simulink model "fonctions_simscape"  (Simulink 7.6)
settings: Solver=ode15s  StartTime=0.0  StopTime=1  RelTol=1e-3
InitFcn:
  | R1=10e3;
  | R2=20e3;
libraries: fl_lib x12, nesl_utility x4, elec_lib x1

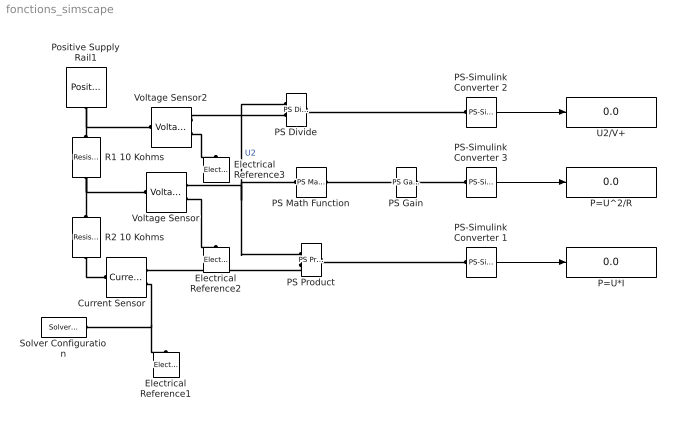
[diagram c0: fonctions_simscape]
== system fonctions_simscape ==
  Current Sensor : fl_lib/Electrical/Electrical Sensors/Current Sensor  DialogController=NetworkEngine.DynNeDlgSource  SystemSampleTime=-1  i1_Log=off  v1_Log=off  LocalVarNames=|i1|v1  LocalVarDescs=|i1|v1  LocalVarLogging=[0 0]
  Electrical Reference1 : fl_lib/Electrical/Electrical Elements/Electrical Reference  DialogController=NetworkEngine.DynNeDlgSource  SystemSampleTime=-1  i_Log=off  LocalVarNames=|i  LocalVarDescs=|i  LocalVarLogging=[]
  Electrical Reference2 : fl_lib/Electrical/Electrical Elements/Electrical Reference  DialogController=NetworkEngine.DynNeDlgSource  SystemSampleTime=-1  i_Log=off  LocalVarNames=|i  LocalVarDescs=|i  LocalVarLogging=[]
  Electrical Reference3 : fl_lib/Electrical/Electrical Elements/Electrical Reference  DialogController=NetworkEngine.DynNeDlgSource  SystemSampleTime=-1  i_Log=off  LocalVarNames=|i  LocalVarDescs=|i  LocalVarLogging=[]
  P=U*I : Display
  P=U^2/R : Display
  PS Divide : fl_lib/Physical Signals/Functions/PS Divide  DialogController=NetworkEngine.DynNeDlgSource  SystemSampleTime=-1  LocalVarLogging=[]
  PS Gain : fl_lib/Physical Signals/Functions/PS Gain  DialogController=NetworkEngine.DynNeDlgSource  SystemSampleTime=-1  gain=1/R2  LocalVarLogging=[]
  PS Math Function : fl_lib/Physical Signals/Functions/PS Math Function  DialogController=NetworkEngine.DynNeDlgSource  SystemSampleTime=-1  fcn_choice=7  LocalVarLogging=[]
  PS Product : fl_lib/Physical Signals/Functions/PS Product  DialogController=NetworkEngine.DynNeDlgSource  SystemSampleTime=-1  LocalVarLogging=[]
  PS-Simulink Converter 1 : nesl_utility/PS-Simulink Converter  DialogController=NetworkEngine.DynNeUtilDlgSource  SystemSampleTime=-1  PhysicalDomain=network_engine_domain  LeftPortType=input  RightPortType=output  SubClassName=ps_output  Unit=W  AffineConversion=off
  PS-Simulink Converter 2 : nesl_utility/PS-Simulink Converter  DialogController=NetworkEngine.DynNeUtilDlgSource  SystemSampleTime=-1  PhysicalDomain=network_engine_domain  LeftPortType=input  RightPortType=output  SubClassName=ps_output  Unit=V  AffineConversion=off
  PS-Simulink Converter 3 : nesl_utility/PS-Simulink Converter  DialogController=NetworkEngine.DynNeUtilDlgSource  SystemSampleTime=-1  PhysicalDomain=network_engine_domain  LeftPortType=input  RightPortType=output  SubClassName=ps_output  Unit=W  AffineConversion=off
  Positive Supply Rail1 : elec_lib/Sources/Positive Supply Rail  DialogController=NetworkEngine.DynNeDlgSource  SystemSampleTime=-1  v0=12 V  current_Log=off  voltage_Log=off  power_Log=off  LocalVarNames=|current|voltage|power  LocalVarDescs=|Current (A)|Voltage (V)|Power (W)  LocalVarLogging=[0 0 0]
  R1 10 Kohms : fl_lib/Electrical/Electrical Elements/Resistor  DialogController=NetworkEngine.DynNeDlgSource  SystemSampleTime=-1  R=R1 Ohm  i_Log=off  v_Log=off  LocalVarNames=|i|v  LocalVarDescs=|i|v  LocalVarLogging=[0 0]
  R2 10 Kohms : fl_lib/Electrical/Electrical Elements/Resistor  DialogController=NetworkEngine.DynNeDlgSource  SystemSampleTime=-1  R=R2 Ohm  i_Log=off  v_Log=off  LocalVarNames=|i|v  LocalVarDescs=|i|v  LocalVarLogging=[0 0]
  Solver Configuration : nesl_utility/Solver Configuration  DialogController=NetworkEngine.DynNeUtilDlgSource  SystemSampleTime=-1  PhysicalDomain=network_engine_domain  LeftPortType=input  RightPortType=generic  SubClassName=solver  Accelerate=off  Profile=off  ResidualTolerance=1e-9  MaxNonlinIter=12  MaxModeIter=2  DoFixedCost=off  UseLocalSampling=off  DoDC=off  LinearAlgebra=Sparse  LocalSolverSampleTime=.001  LocalSolverChoice=NE_BACKWARD_EULER_ADVANCER  UseLocalSolver=off
  U2/V+ : Display
  Voltage Sensor2 : fl_lib/Electrical/Electrical Sensors/Voltage Sensor  DialogController=NetworkEngine.DynNeDlgSource  SystemSampleTime=-1  i1_Log=off  v1_Log=off  LocalVarNames=|i1|v1  LocalVarDescs=|i1|v1  LocalVarLogging=[]
  Voltage Sensor : fl_lib/Electrical/Electrical Sensors/Voltage Sensor  DialogController=NetworkEngine.DynNeDlgSource  SystemSampleTime=-1  i1_Log=off  v1_Log=off  LocalVarNames=|i1|v1  LocalVarDescs=|i1|v1  LocalVarLogging=[0 0]
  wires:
  PS-Simulink Converter 3/1 -> P=U^2/R/1
  PS-Simulink Converter 1/1 -> P=U*I/1
  PS-Simulink Converter 2/1 -> U2/V+/1
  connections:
  Positive Supply Rail1/RConn1 -- R1 10 Kohms/LConn1 -- Voltage Sensor2/LConn1
  R1 10 Kohms/RConn1 -- R2 10 Kohms/LConn1 -- Voltage Sensor/LConn1
  Voltage Sensor/RConn2 -- Electrical Reference2/LConn1
  Voltage Sensor/RConn1 -- PS Math Function/LConn1 -- PS Product/LConn1 -- PS Divide/LConn1  "U2"
  PS Math Function/RConn1 -- PS Gain/LConn1
  PS Gain/RConn1 -- PS-Simulink Converter 3/LConn1
  R2 10 Kohms/RConn1 -- Current Sensor/LConn1
  Current Sensor/RConn2 -- Solver Configuration/RConn1 -- Electrical Reference1/LConn1
  PS Product/LConn2 -- Current Sensor/RConn1
  PS Product/RConn1 -- PS-Simulink Converter 1/LConn1
  Voltage Sensor2/RConn2 -- Electrical Reference3/LConn1
  PS Divide/RConn1 -- PS-Simulink Converter 2/LConn1
  Voltage Sensor2/RConn1 -- PS Divide/LConn2
